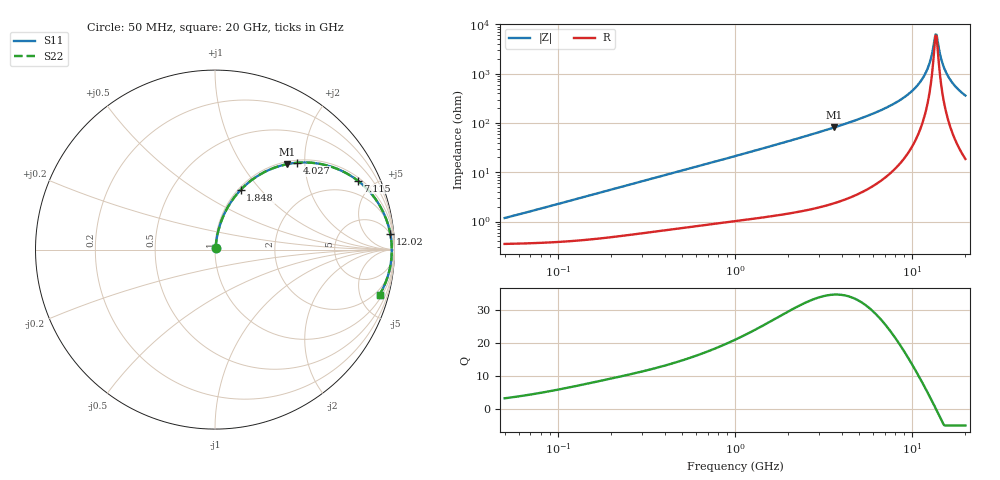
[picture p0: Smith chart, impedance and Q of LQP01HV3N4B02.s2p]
!Murata Part Number: LQP01HV3N4B02
!These Parameters are Measured in Series Mode Connection
!  o--[Z]--o
!Port1  Port2
!  o-------o
!Freq. Start=50[MHz] Stop=20[GHz], 401[Steps]
# Hz S RI R 50
!Freq.(Hz) S11(Real) S11(Imag) S21(Real) S21(Imag) S12(Real) S12(Imag) S22(Real) S22(Imag)
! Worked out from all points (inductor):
!   401 points, 50 MHz to 20 GHz, reference 50 ohm
!   read as one part in series: L = 3.58 nH near 51.52 MHz
!   highest Q = 34.5 at 3.626 GHz (marker M1), where L = 3.56 nH
!   self-resonance near 13.55 GHz
!   S11 on the Smith chart (normalised r, x): 50 MHz: 1.01, +0.02; 1.848 GHz: 1.03, +0.79; 4.027 GHz: 1.05, +1.83; 7.115 GHz: 1.16, +4.05; 12.02 GHz: 5, +22; 20 GHz: 1.37, -7.21
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5e7  0.00363 0.0112  0.9964 -0.0112  0.9964 -0.0112  0.00363 0.0112
1.364002e8  0.00508 0.0302  0.9949 -0.0302  0.9949 -0.0302  0.00508 0.0302
3.721004e8  0.0127 0.0793  0.9873 -0.0793  0.9873 -0.0793  0.0127 0.0793
1e9  0.052 0.1994  0.948 -0.1994  0.948 -0.1994  0.052 0.1994
1.848039e9  0.143 0.3329  0.857 -0.3329  0.857 -0.3329  0.143 0.3329
2.728004e9  0.266 0.427  0.734 -0.427  0.734 -0.427  0.266 0.427
3.626126e9  0.4001 0.4757  0.5999 -0.4757  0.5999 -0.4757  0.4001 0.4757
4.026975e9  0.4583 0.4839  0.5417 -0.4839  0.5417 -0.4839  0.4583 0.4839
5.352748e9  0.6294 0.4674  0.3706 -0.4674  0.3706 -0.4674  0.6294 0.4674
7.114996e9  0.7952 0.3842  0.2048 -0.3842  0.2048 -0.3842  0.7952 0.3842
7.442007e9  0.8186 0.365  0.1814 -0.365  0.1814 -0.365  0.8186 0.365
1.004137e10  0.9398 0.2032  0.0602 -0.2032  0.0602 -0.2032  0.9398 0.2032
1.115139e10  0.965 0.1362  0.035 -0.1362  0.035 -0.1362  0.965 0.1362
1.201863e10  0.977 0.0863  0.023 -0.0863  0.023 -0.0863  0.977 0.0863
1.257102e10  0.9816 0.0559  0.0184 -0.0559  0.0184 -0.0559  0.9816 0.0559
1.334722e10  0.9847 0.015  0.0153 -0.015  0.0153 -0.015  0.9847 0.015
1.375312e10  0.985 -0.00552  0.015 0.00552  0.015 0.00552  0.985 -0.00552
1.396067e10  0.9849 -0.0158  0.0151 0.0158  0.0151 0.0158  0.9849 -0.0158
1.482269e10  0.982 -0.0567  0.018 0.0567  0.018 0.0567  0.982 -0.0567
1.573793e10  0.9757 -0.0973  0.0243 0.0973  0.0243 0.0973  0.9757 -0.0973
1.747767e10  0.9566 -0.1666  0.0434 0.1666  0.0434 0.1666  0.9566 -0.1666
2e10  0.9176 -0.2504  0.0824 0.2504  0.0824 0.2504  0.9176 -0.2504
